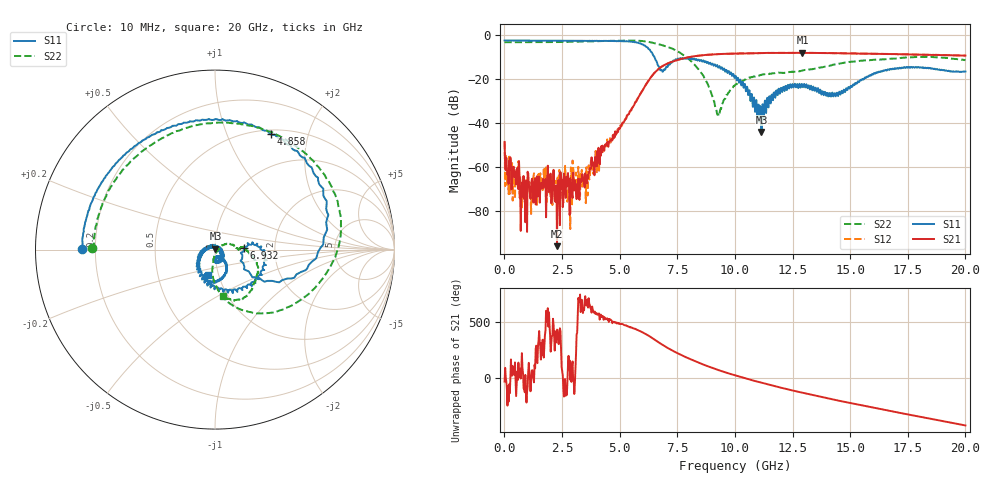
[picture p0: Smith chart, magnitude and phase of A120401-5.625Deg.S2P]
!  2-Port S-parameters saved by WinCal
! VAR MeasName=S-Parameters (CALIBRATED_DATA) read from VNA (N5244A)
! VAR MeasDate=11/21/2012 9:55:23 AM
! VAR NAME=A120401-5.625Deg
! VAR FILENAME=A120401-5.625Deg.S2P
! VAR DATE=11/21/2012 9:55:23 AM
! VAR PHYS_PORTS=1,2
# Hz S MA R 50
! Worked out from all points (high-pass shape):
!   801 points, 10 MHz to 20 GHz, reference 50 ohm
!   highest |S21| = -8.22 dB at 12.93 GHz (marker M1); lowest = -96.2 dB at 2.284 GHz (marker M2)
!   |S21| within 3 dB of the highest: 7.594 GHz to end of sweep
!   lowest |S11| = -44.2 dB at 11.15 GHz (marker M3), VSWR 1.01, Z = 50.2 + j0.57 ohm
!   |S11| at or under -10 dB: 6.506 GHz to end of sweep
!   |S22| runs from -36.9 to -2.6 dB; largest |S21 - S12| = 0.0043
!   S11 on the Smith chart (normalised r, x): 10 MHz: 0.15, +0.00; 4.858 GHz: 0.55, +1.44; 6.932 GHz: 1.39, +0.02; 20 GHz: 0.89, -0.26
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1e7  0.7417 179.7  0.00366 -36.0  0.003715 -44.8  0.6834 179.3
1.349375e8  0.7383 177.4  0.0006489 105.7  0.0007151 -179.2  0.6762 176.7
5.847125e8  0.7384 168.8  0.0008984 -21.1  0.0008807 92.0  0.676 165.8
8.096e8  0.7371 164.5  0.0002049 39.5  0.000593 -83.9  0.6758 160.5
1.10945e9  0.7352 158.5  0.0002459 -4.8  0.0002086 13.2  0.6772 153.3
2.283862e9  0.7298 134.8  1.553e-05 74.9  0.000282 7.6  0.682 124.7
2.833588e9  0.728 122.8  7.921e-05 154.8  0.0001135 86.6  0.6903 111.0
3.358325e9  0.7249 109.9  0.0004675 -14.0  0.0008428 12.5  0.7008 97.8
4.857575e9  0.714 64.3  0.005636 138.6  0.005566 141.5  0.7297 54.6
5.882062e9  0.636 11.5  0.04359 62.0  0.04437 63.1  0.7273 17.4
6.681662e9  0.1945 -34.0  0.1656 -38.9  0.1655 -38.9  0.6099 -17.7
6.931538e9  0.1624 2.5  0.2029 -72.4  0.2028 -72.0  0.5617 -28.8
8.430788e9  0.2726 -55.8  0.3352 134.8  0.3332 134.8  0.1616 -93.5
9.255375e9  0.1923 -100.0  0.3618 70.7  0.3612 70.7  0.01575 -44.0
1.0005e10  0.1081 -151.3  0.3719 20.5  0.3738 20.5  0.07118 27.3
1.115442e10  0.006178 66.6  0.384 -46.6  0.3834 -46.7  0.1223 3.6
1.187906e10  0.05598 -42.9  0.3861 -85.5  0.3883 -85.4  0.1375 2.0
1.292854e10  0.06825 -75.9  0.3884 -137.3  0.3878 -137.5  0.1539 4.7
1.335332e10  0.05445 -91.2  0.386 -157.4  0.3867 -157.5  0.1645 1.8
1.437781e10  0.03977 -69.0  0.3805 156.1  0.3822 156.0  0.2136 -10.4
1.667666e10  0.1603 -73.6  0.3642 59.3  0.3644 59.2  0.2831 -36.5
2e10  0.1454 -104.8  0.3351 -74.1  0.3341 -74.2  0.2637 -80.1
